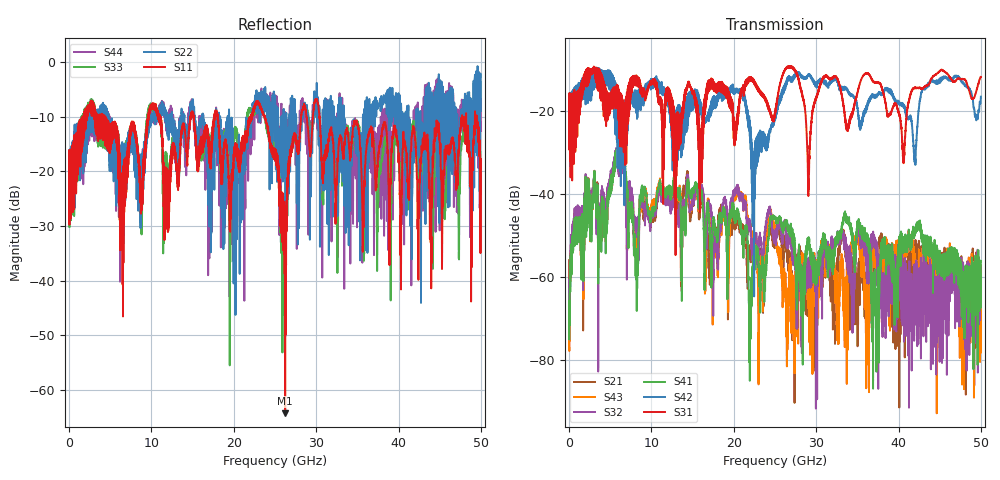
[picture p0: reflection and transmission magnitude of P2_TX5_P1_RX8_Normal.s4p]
!Keysight Technologies,N5225B,MY57041031,A.13.20.10
!Date: Friday, May 31, 2019 11:26:56
!Correction: S11(Full 4 Port(1,2,3,4))
!S12(Full 4 Port(1,2,3,4))
!S13(Full 4 Port(1,2,3,4))
!S14(Full 4 Port(1,2,3,4))
!S21(Full 4 Port(1,2,3,4))
!S22(Full 4 Port(1,2,3,4))
!S23(Full 4 Port(1,2,3,4))
!S24(Full 4 Port(1,2,3,4))
!S31(Full 4 Port(1,2,3,4))
!S32(Full 4 Port(1,2,3,4))
!S33(Full 4 Port(1,2,3,4))
!S34(Full 4 Port(1,2,3,4))
!S41(Full 4 Port(1,2,3,4))
!S42(Full 4 Port(1,2,3,4))
!S43(Full 4 Port(1,2,3,4))
!S44(Full 4 Port(1,2,3,4))
!S4P File: Measurements: <S11,S12,S13,S14>,
!<S21,S22,S23,S24>,
!<S31,S32,S33,S34>,
!<S41,S42,S43,S44>:
# Hz S  dB  R 50.0
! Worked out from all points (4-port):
!   5000 points, 10 MHz to 50 GHz, reference 50 ohm
!   strongest paths, dB at 10 MHz, 12.51 GHz, 25.01 GHz, 37.51 GHz, 50 GHz:
!     S31: -19.5, -17.8, -20.9, -13.2, -11.7
!     S42: -19.4, -24.2, -22.2, -15.9, -16.5
!     S41: -65.8, -38.7, -45.7, -73.3, -56.3
!     S32: -60.9, -42.0, -50.6, -57.1, -61.6
!     S43: -67.6, -39.1, -48.8, -54.4, -62.5
!     S21: -56.0, -40.3, -51.8, -55.0, -65.5
!   lowest |S11| = -64.3 dB at 26.24 GHz (marker M1), VSWR 1.00, Z = 49.9 + j0.0112 ohm
!   |S11| at or under -10 dB: 4.282 GHz to 9.568 GHz (5.286 GHz wide, 76.3 % of centre); 23.74 GHz to 28.18 GHz (4.439 GHz wide, 17.1 % of centre); 30.41 GHz to 47.7 GHz (17.29 GHz wide, 44.3 % of centre)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
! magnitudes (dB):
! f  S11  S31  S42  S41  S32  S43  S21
! 10 MHz  -19.8  -19.5  -19.4  -65.8  -60.9  -67.6  -56.0
! 5.85 GHz  -14.9  -18.9  -27.4  -31.1  -31.3  -31.3  -31.2
! 8.14 GHz  -13.9  -12.9  -17.0  -55.1  -45.9  -49.8  -49.8
! 22.93 GHz  -7.1  -14.9  -27.9  -55.1  -55.3  -59.5  -57.2
! 26.24 GHz  -64.3  -9.9  -14.3  -47.2  -46.8  -63.5  -50.5
! 30.01 GHz  -6.8  -16.7  -13.5  -61.4  -74.1  -60.2  -71.4
! 50 GHz  -19.5  -11.7  -16.5  -56.3  -61.6  -62.5  -65.5
